(* Logix 5000 AddOnInstructionDefinition export AMCI_SD4840E2_Preset_Encoder_Position; software revision 20.03 *)

ADD_ON_INSTRUCTION AMCI_SD4840E2_Preset_Encoder_Position   (* revision 1.0, vendor AMCI *)
VAR_INPUT
   Target_Position : DINT; {required}
END_VAR
VAR_IN_OUT
   AMCI_SD4840E2_output_data : _000A:SD4840E2_4342D302:O:0; {required}
END_VAR
VAR
   Upper_Result_X_1000 : DINT;
   command_data_block : INT[10];
        [0]   // Command Bits MSW
        [1]   // Command Bits LSW
        [2]   // Upper Target Position
        [3]   // Lower Target Position
        [4]   // Upper Programmed Speed
        [5]   // Lower Programmed Speed
END_VAR

ROUTINE Logic   (* ladder *)
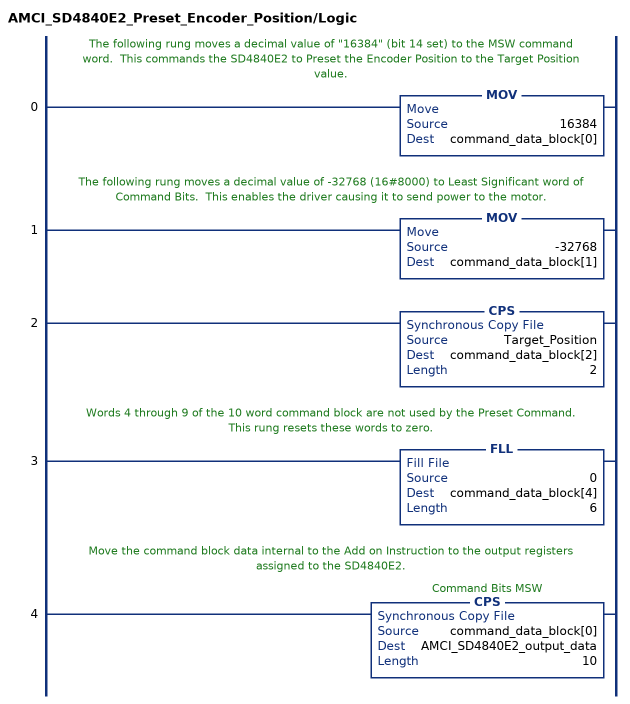
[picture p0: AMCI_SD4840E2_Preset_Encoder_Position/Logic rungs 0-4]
   // The following rung moves a decimal value of "16384" (bit 14 set) to the MSW command word.  This commands the SD4840E2 to Preset the Encoder Position to the Target Position value.
   0: MOV(16384,command_data_block[0]);
   // The following rung moves a decimal value of -32768 (16#8000) to Least Significant word of Command Bits.  This enables the driver causing it to send power to the motor.
   1: MOV(-32768,command_data_block[1]);
   2: CPS(Target_Position,command_data_block[2],2);
   // Words 4 through 9 of the 10 word command block are not used by the Preset Command.  This rung resets these words to zero.
   3: FLL(0,command_data_block[4],6);
   // Move the command block data internal to the Add on Instruction to the output registers assigned to the SD4840E2.
   4: CPS(command_data_block[0],AMCI_SD4840E2_output_data,10);
END_ROUTINE
END_ADD_ON_INSTRUCTION
